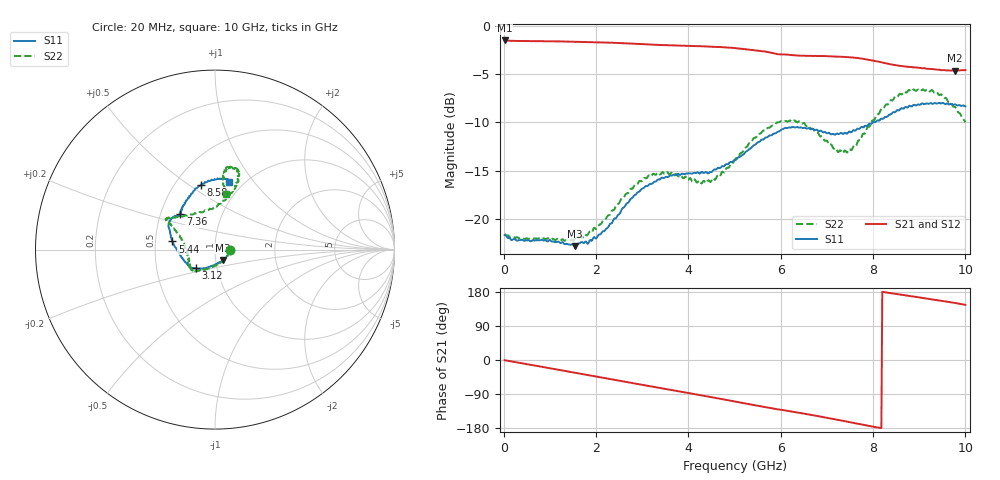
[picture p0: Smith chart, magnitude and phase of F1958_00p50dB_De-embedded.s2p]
! Integrated Device Technology
! Corporate Headquarters
! 6024 Silver Creek Valley Road
! San Jose, CA 95138  USA
! Phone:  1-408-284-8200
! Toll Free:  1-800-223-1366
! Webpage:  http://www.idt.com/
! Timing and RF Division
! 515 Groton Road, Suite 102
! Westford, MA 01886-6024
! Device:  F1958
! Description: 7-bit 0.25 dB Digital Step Attenuator
! Frequency:  0.001 -  6.000 GHz
! Package:  4x4 mm Thin QFN Plastic Package: 24 pin
! Ports:  2 RF, 12 DC
!  Pin  1  = D0
!  Pin  2  = VDD
!  Pin  3  = VMODE
!  Pin  4  = GND
!  Pin  5  = RF1  =  Port 1
!  Pin  6  = GND
!  Pin  7  = GND
!  Pin  8  = GND
!  Pin  9  = GND
!  Pin 10  = GND
!  Pin 11  = GND
!  Pin 12  = GND
!  Pin 13  = GND
!  Pin 14  = RF2  =  Port 2
!  Pin 15  = GND
!  Pin 16  = LE
!  Pin 17  = CLK
!  Pin 18  = DATA
!  Pin 19  = D6
!  Pin 20  = D5
!  Pin 21  = D4
!  Pin 22  = D3
!  Pin 23  = D2
!  Pin 24  = D1
! State:  2
! Atten State:  0.50 dB
! Voltage:  +3.30 Volts
! Current:  0.257 mA
! Data:  The device was measured on a F1958 evaluation board which has
!  individual transmission lines to the RF pins.  Data was collected
!  using a calibrated network analyzer.  The evaluation board was
!  de-embedded using Automatic Fixture Removal (AFR).
!  The reference plane is the edge of the package pin.
! Misc:
!  Action Tracker AT0419
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# GHz S dB R 50
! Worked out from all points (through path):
!   500 points, 20 MHz to 10 GHz, reference 50 ohm
!   highest |S21| = -1.47 dB at 20 MHz (marker M1); lowest = -4.6 dB at 9.78 GHz (marker M2)
!   group delay of S21, straight-line fit = 60.2 ps
!   lowest |S11| = -22.9 dB at 1.54 GHz (marker M3), VSWR 1.16, Z = 54 - j6.33 ohm
!   |S11| at or under -10 dB: start of sweep to 7.992 GHz
!   |S22| runs from -22.3 to -6.5 dB; largest |S21 - S12| = 0.0023
!   S11 on the Smith chart (normalised r, x): 20 MHz: 1.18, -0.01; 3.12 GHz: 0.79, -0.17; 5.44 GHz: 0.61, +0.06; 7.36 GHz: 0.63, +0.27; 8.58 GHz: 0.67, +0.56; 10 GHz: 0.86, +0.76
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0.02  -21.70 -1.9  -1.47 -0.6  -1.47 -0.6  -21.60 -2.1
0.8  -22.23 -19.5  -1.55 -17.4  -1.55 -17.4  -22.11 -23.2
1.54  -22.86 -54.1  -1.61 -33.5  -1.61 -33.5  -22.10 -61.7
1.7  -22.43 -63.5  -1.62 -36.9  -1.62 -36.9  -21.99 -71.1
2.22  -21.05 -96.5  -1.69 -48.3  -1.68 -48.3  -19.95 -100.9
2.78  -17.86 -124.5  -1.80 -60.7  -1.79 -60.7  -16.91 -124.8
3.12  -16.59 -135.1  -1.88 -68.1  -1.88 -68.2  -15.62 -134.8
3.36  -15.93 -139.1  -1.94 -73.3  -1.94 -73.4  -15.29 -138.3
4.42  -15.30 -154.0  -2.10 -96.4  -2.11 -96.4  -16.04 -173.1
5.02  -13.90 -174.5  -2.27 -109.9  -2.28 -109.9  -13.76 160.8
5.44  -12.32 169.2  -2.50 -119.3  -2.51 -119.4  -11.58 152.8
5.98  -10.88 154.3  -2.92 -130.8  -2.93 -130.7  -9.92 148.5
6.38  -10.51 145.5  -3.04 -139.0  -3.06 -139.0  -9.93 146.3
6.68  -10.66 140.8  -3.08 -145.2  -3.10 -145.2  -10.65 141.7
7.36  -11.17 134.5  -3.18 -160.9  -3.19 -160.8  -13.09 105.8
7.6  -10.85 131.6  -3.27 -166.5  -3.27 -166.4  -12.39 90.9
8.02  -9.95 120.6  -3.59 -176.4  -3.60 -176.4  -9.78 74.7
8.34  -9.22 110.6  -3.91 177.2  -3.91 177.1  -8.02 71.1
8.58  -8.67 102.1  -4.11 172.7  -4.11 172.8  -7.01 73.0
9.26  -8.00 84.1  -4.45 160.2  -4.45 160.1  -6.66 80.6
9.78  -8.12 78.1  -4.61 150.3  -4.63 150.4  -8.40 82.5
10  -8.32 78.1  -4.55 145.4  -4.58 145.5  -9.98 79.0
